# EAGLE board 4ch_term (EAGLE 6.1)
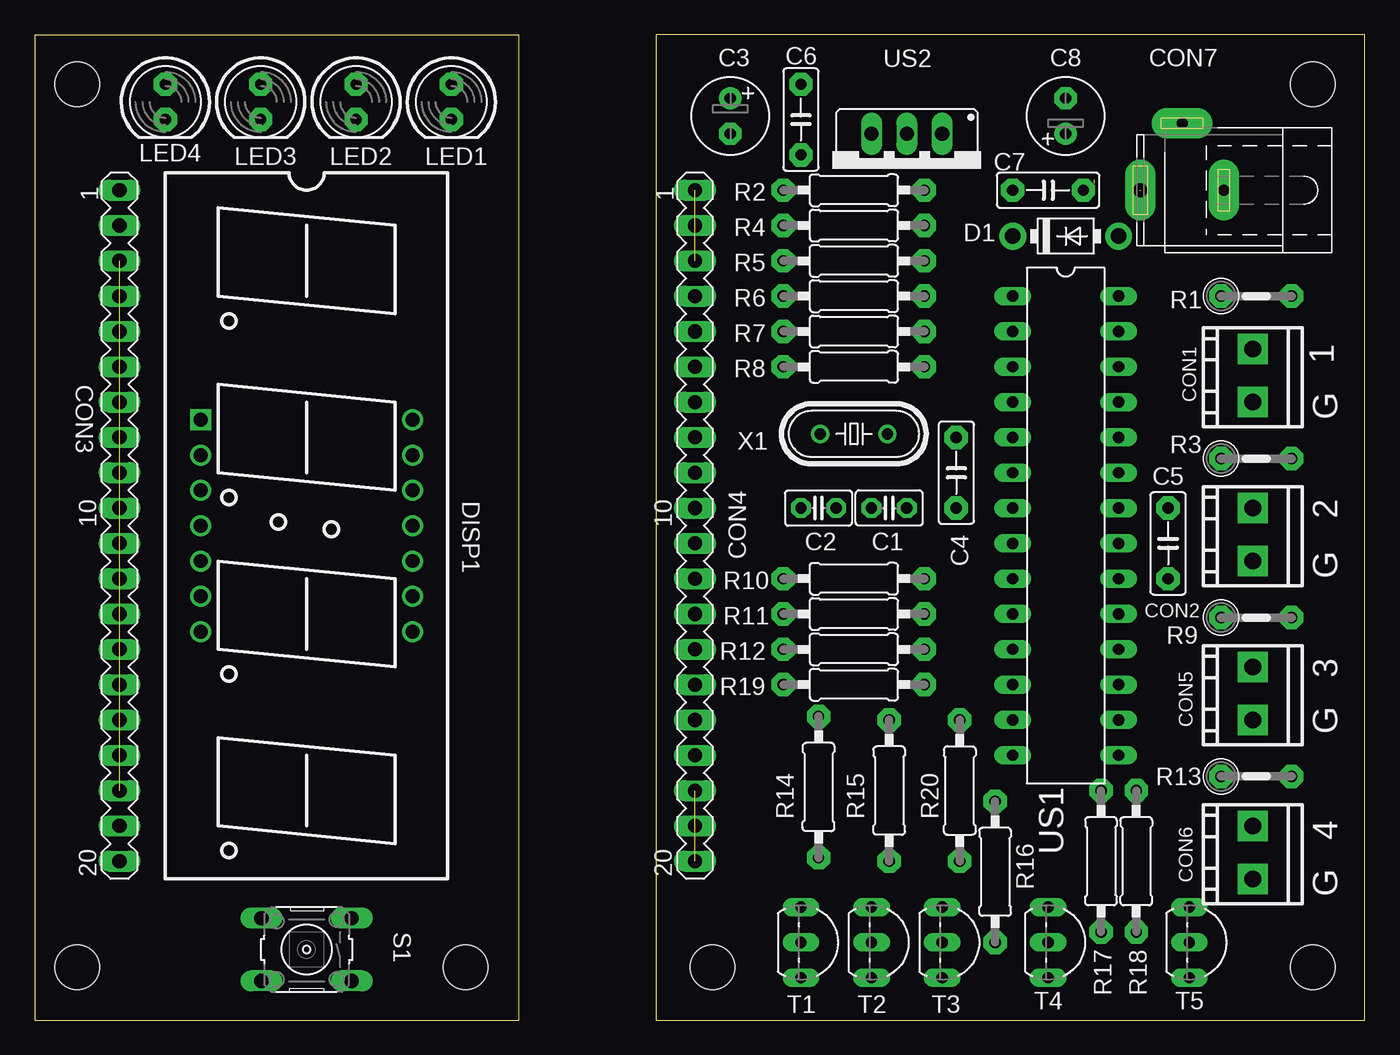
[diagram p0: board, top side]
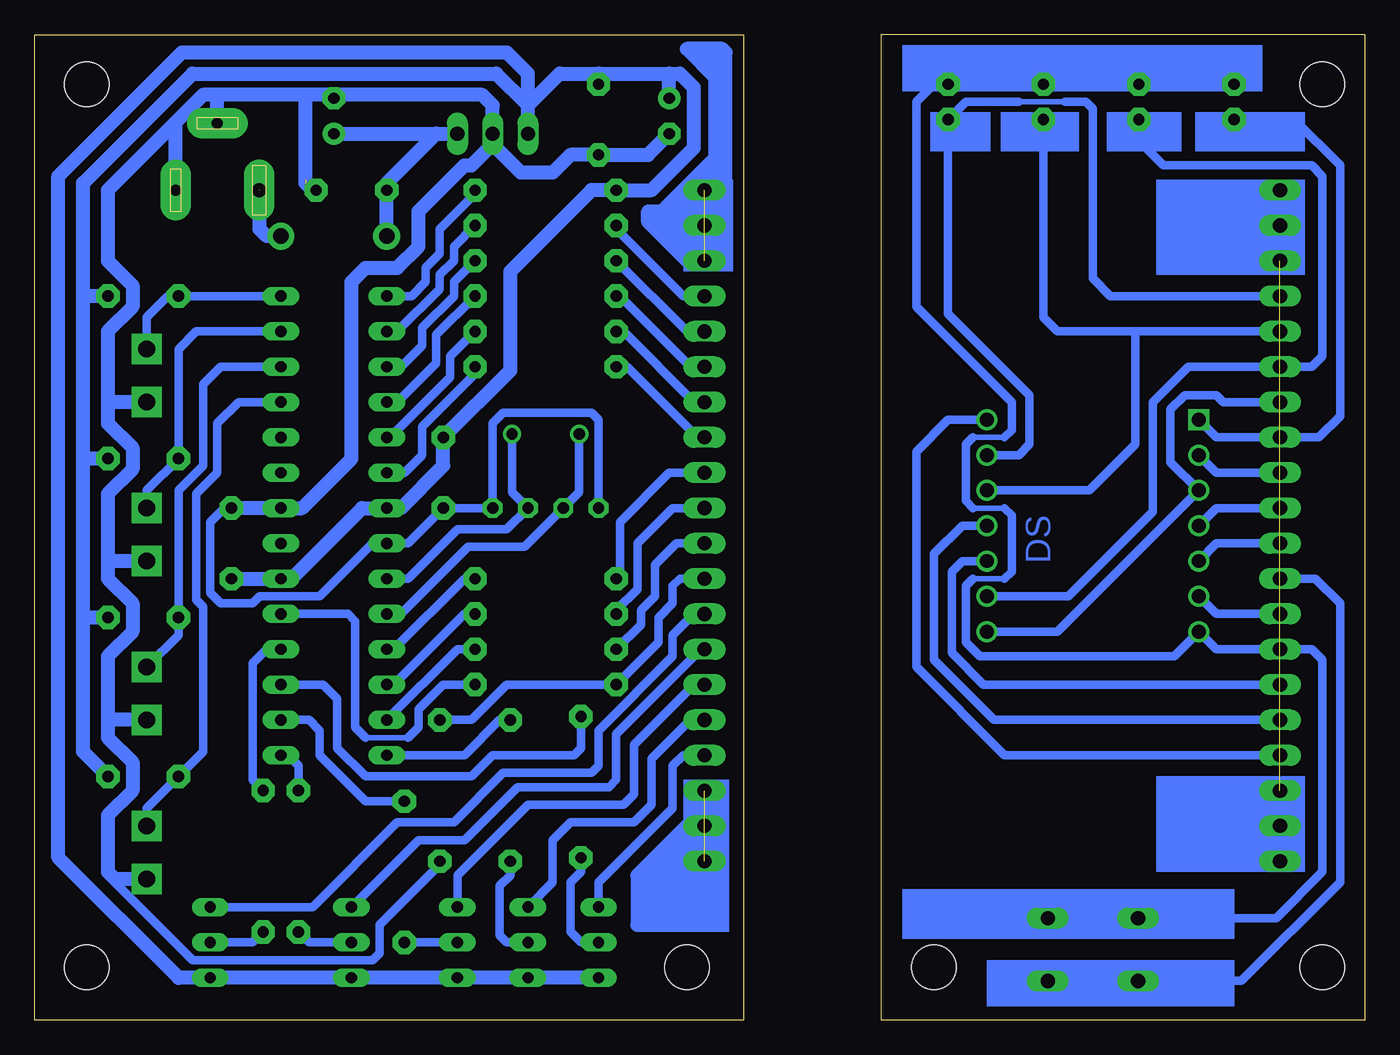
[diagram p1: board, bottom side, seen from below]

Size 95.68 x 70.87 mm. Coordinates in mm from the lower left corner, seen from the top.
Outline: 0,70.86 0,0 34.8,0 34.8,70.86
Outline: 0.01,70.87 34.8,70.87
Outline: 44.7,0 95.68,0 95.68,70.86 44.7,70.86 44.7,0
Copper layers (1*16): Top 0.035mm / dielectric 1.5mm / Bottom 0.035mm
Design rules: minimum track width 10mil, minimum drill 24mil, track to track 8mil, track to pad 8mil, pad to pad 8mil, via to via 8mil, smd to smd 8mil, copper to edge 40mil, drill to drill 8mil, minimum pad ring 10mil, minimum via ring 8mil, stop-mask expansion 4mil, vias tented up to drill 0mil, thermal gap 10mil
Holes 3.2 mm at 91.95,3.81 91.95,67.31 48.77,3.81 3.05,67.31 3.05,3.81 30.99,3.81

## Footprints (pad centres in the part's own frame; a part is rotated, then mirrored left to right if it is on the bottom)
C025-025X050 = drill 0.813 pad 1.422 octagon: 1 -1.27,0; 2 1.27,0
E2,5-6 = drill 0.813 pad 1.6: + -1.27,0 | drill 0.813 pad 1.6 octagon: - 1.27,0
C050-025X075 = drill 0.813 pad 1.676 octagon: 1 -2.54,0; 2 2.54,0
ARK2/300 = drill 1.2 pad 2.184 square: 1 -2.54,0; 2 1.27,0
MA20-1 = drill 1.016 long: 1 -24.13,0; 2 -21.59,0; 3 -19.05,0; 4 -16.51,0; 5 -13.97,0; 6 -11.43,0; 7 -8.89,0; 8 -6.35,0; 9 -3.81,0; 10 -1.27,0; 11 1.27,0; 12 3.81,0; 13 6.35,0; 14 8.89,0; 15 11.43,0; 16 13.97,0; 17 16.51,0; 18 19.05,0; 19 21.59,0; 20 24.13,0
SPC4077 = drill 0.8 pad 2.184 long: 1 -3,0; 2 0,-4.8 | drill 1 pad 2.184 long: 3 3,0
DO41-10 = drill 1.118 pad 1.93: A 3.81,0; C -3.81,0
DISP7X4 = drill 1 square: 1 -7.62,-7.62 | drill 1: 2 -5.08,-7.62; 3 -2.54,-7.62; 4 0,-7.62; 5 2.54,-7.62; 6 5.08,-7.62; 7 7.62,-7.62; 8 7.62,7.62; 9 5.08,7.62; 10 2.54,7.62; 11 0,7.62; 12 -2.54,7.62; 13 -5.08,7.62; 14 -7.62,7.62
LED5MM = drill 0.813 pad 1.676 octagon: A -1.27,0; K 1.27,0
0207/5V = drill 0.813 pad 1.676 octagon: 1 -2.54,0; 2 2.54,0
0207/10 = drill 0.813 pad 1.676 octagon: 1 -5.08,0; 2 5.08,0
B3F-10XX = drill 1.016 long: 1 -3.251,2.261; 2 3.251,2.261; 3 -3.251,-2.261; 4 3.251,-2.261
TO92-EBC = drill 0.813 long: B 0,-1.27; C -2.54,-1.27; E 2.54,-1.27
DIL28-3 = drill 0.813 long: 1 -16.51,-3.81; 2 -13.97,-3.81; 3 -11.43,-3.81; 4 -8.89,-3.81; 5 -6.35,-3.81; 6 -3.81,-3.81; 7 -1.27,-3.81; 8 1.27,-3.81; 9 3.81,-3.81; 10 6.35,-3.81; 11 8.89,-3.81; 12 11.43,-3.81; 13 13.97,-3.81; 14 16.51,-3.81; 15 16.51,3.81; 16 13.97,3.81; 17 11.43,3.81; 18 8.89,3.81; 19 6.35,3.81; 20 3.81,3.81; 21 1.27,3.81; 22 -1.27,3.81; 23 -3.81,3.81; 24 -6.35,3.81; 25 -8.89,3.81; 26 -11.43,3.81; 27 -13.97,3.81; 28 -16.51,3.81
78XXS = drill 1.016 long: GND 0,-2.54; IN -2.54,-2.54; OUT 2.54,-2.54
HC49/S = drill 0.813: 1 -2.413,0; 2 2.413,0

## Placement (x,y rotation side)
C1  [C025-025X050]  61.47,36.83 180 top
C2  [C025-025X050]  56.39,36.83 0 top
C3  220uF  [E2,5-6]  50.04,65.02 270 top
C4  100n  [C050-025X075]  66.29,39.37 270 top
C5  100n  [C050-025X075]  81.53,34.29 90 top
C6  100n  [C050-025X075]  55.12,64.77 270 top
C7  100n  [C050-025X075]  72.9,59.69 0 top
C8  220uF  [E2,5-6]  74.17,65.02 90 top
CON1  [ARK2/300]  87.63,46.99 90 top
CON2  [ARK2/300]  87.63,35.56 90 top
CON3  [MA20-1]  6.1,35.56 270 top
CON4  [MA20-1]  47.5,35.56 270 top
CON5  [ARK2/300]  87.63,24.13 90 top
CON6  [ARK2/300]  87.63,12.7 90 top
CON7  [SPC4077]  82.55,59.69 180 top
D1  1N4004  [DO41-10]  74.17,56.39 0 top
DISP1  DISP7X4  [DISP7X4]  19.56,35.56 270 top
LED1  [LED5MM]  29.97,66.04 270 top
LED2  [LED5MM]  23.11,66.04 270 top
LED3  [LED5MM]  16.26,66.04 270 top
LED4  [LED5MM]  9.4,66.04 270 top
R1  4.7k  [0207/5V]  87.88,52.07 0 top
R2  [0207/10]  58.93,59.69 0 top
R3  4.7k  [0207/5V]  87.88,40.39 0 top
R4  [0207/10]  58.93,57.15 0 top
R5  [0207/10]  58.93,54.61 0 top
R6  [0207/10]  58.93,52.07 0 top
R7  [0207/10]  58.93,49.53 0 top
R8  [0207/10]  58.93,46.99 0 top
R9  4.7k  [0207/5V]  87.88,28.96 0 top
R10  [0207/10]  58.93,31.75 0 top
R11  [0207/10]  58.93,29.21 0 top
R12  [0207/10]  58.93,26.67 0 top
R13  4.7k  [0207/5V]  87.88,17.53 0 top
R14  [0207/10]  56.39,16.76 90 top
R15  [0207/10]  61.47,16.51 90 top
R16  [0207/10]  69.09,10.67 90 top
R17  [0207/10]  76.71,11.43 90 top
R18  [0207/10]  79.25,11.43 90 top
R19  [0207/10]  58.93,24.13 0 top
R20  [0207/10]  66.55,16.51 270 top
S1  [B3F-10XX]  19.56,5.08 180 top
T1  [TO92-EBC]  56.39,5.59 270 top
T2  [TO92-EBC]  61.47,5.59 270 top
T3  [TO92-EBC]  66.55,5.59 270 top
T4  [TO92-EBC]  74.17,5.59 270 top
T5  [TO92-EBC]  84.33,5.59 270 top
US1  ATMEGA8  [DIL28-3]  74.17,35.56 270 top
US2  7805  [78XXS]  62.74,61.21 180 top
X1  8MHz  [HC49/S]  58.93,42.16 0 top

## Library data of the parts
C1-C8 R1-R20 = rcl
CON1 CON2 CON5 CON6 DISP1 = ds_lib_eagle
CON3 CON4 = con-lstb; OC_FARNELL: unknown; OC_NEWARK: unknown
CON7 = con-jack; OC_FARNELL: unknown; OC_NEWARK: unknown
D1 = diode
LED1-LED4 = led
S1 = switch-omron; MPN: B3F-1000; OC_FARNELL: 176432; OC_NEWARK: 36M3542
T1-T5 = transistor-pnp
US1 = avr-4
US2 = v-reg
X1 = crystal; OC_FARNELL: 1667008; OC_NEWARK: unknown

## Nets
+5V: C3.+ C4.1 C5.1 C6.1 R1.2 R2.1 R3.2 R9.2 R13.2 T1.E T2.E T3.E T4.E T5.E US1.7 US1.20 US2.OUT
A: CON3.4 DISP1.13 LED1.K
A1: CON3.17 DISP1.14
A2: CON3.16 DISP1.11
A3: CON3.15 DISP1.10
A4: CON3.13 DISP1.6
A5: CON3.14 DISP1.7 LED1.A LED2.A LED3.A LED4.A S1.4
B: CON3.6 DISP1.9 LED3.K
C: CON3.10 DISP1.4
D: CON3.9 DISP1.2
DP: CON3.7 DISP1.3 DISP1.8
E: CON3.8 DISP1.1 LED4.K
F: CON3.5 DISP1.12 LED2.K
G: CON3.11 DISP1.5
GND: C1.1 C2.1 C3.- C4.2 C5.2 C6.2 C7.2 C8.- CON1.1 CON2.1 CON5.1 CON6.1 CON7.1 CON7.2 R20.2 US1.8 US1.22 US2.GND
N$1: CON4.4 R4.1
N$2: CON4.5 R5.1
N$3: CON4.6 R6.1
N$4: CON4.7 R7.1
N$5: CON4.8 R8.1
N$6: CON4.9 R10.1
N$7: CON4.10 R11.1
N$8: CON4.11 R12.1
N$9: CON4.13 T5.C
N$10: CON4.14 T4.C
N$11: CON4.15 T3.C
N$12: CON4.16 T2.C
N$13: CON4.17 T1.C
N$14: R14.1 T1.B
N$15: R15.1 T2.B
N$16: R16.1 T3.B
N$17: R18.1 T5.B
N$18: R17.1 T4.B
N$19: CON4.12 R19.1 R20.1
N$20: C7.1 C8.+ D1.C US2.IN
N$21: C1.2 US1.9 X1.2
N$22: C2.2 US1.10 X1.1
N$23: R2.2 US1.1
N$24: CON7.3 D1.A
N$33: US1.23
N$34: CON4.18 CON4.19 CON4.20
N$35: CON4.1 CON4.2 CON4.3
N$36: US1.24
NC: CON3.1 CON3.2 CON3.3 CON3.18 CON3.19 CON3.20
SA: R4.2 US1.2
SB: R5.2 US1.3
SC: R6.2 US1.4
SD: R7.2 US1.5
SDP: R12.2 US1.13
SE: R8.2 US1.6
SF: R10.2 US1.11
SG: R11.2 US1.12
SSW: R19.2 US1.19
SW: CON3.12 S1.2
TA1: R15.2 US1.14
TA2: R17.2 US1.15
TA3: R16.2 US1.16
TA4: R14.2 US1.17
TA5: R18.2 US1.18
TR1: CON1.2 R1.1 US1.28
TR2: CON2.2 R3.1 US1.27
TR3: CON5.2 R9.1 US1.26
TR4: CON6.2 R13.1 US1.25

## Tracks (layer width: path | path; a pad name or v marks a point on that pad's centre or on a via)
+5V
  Bottom 1.016: T1.E T2.E | T2.E 60.45,3.05 | T2.E T3.E T4.E T5.E 85.34,3.05 93.98,11.68 93.98,60.71 85.09,69.6 61.72,69.6 60.2,68.07 US2.OUT 60.2,65.79 | 60.2,65.79 62.48,68.07 84.33,68.07 92.2,60.2 92.2,52.07 | 60.2,65.79 57.91,68.07 55.12,68.07 | 55.12,68.07 50.04,68.07 | 50.04,68.07 49.28,68.07 48.26,67.06 48.26,62.74 51.31,59.69 R2.1 55.63,59.69 61.47,53.85 61.47,46.74 C4.1 66.29,39.88 69.34,36.83 US1.7 72.14,36.83 77.22,31.75 US1.20 C5.1 | C3.+ 50.04,68.07 | C6.1 55.12,68.07 | R1.2 92.2,52.07 | R13.2 92.2,19.3 92.2,28.7 | 92.2,28.7 92.2,40.39 | 92.2,40.39 92.2,52.07 | R3.2 92.2,40.39 | R9.2 91.95,28.96 92.2,28.7
A
  Bottom 0.406: 21.59,66.04 24.89,66.04
  Bottom 0.61: DISP1.13 24.89,40.64 24.13,41.4 24.13,44.96 29.97,50.8 LED1.K 28.7,66.04 24.89,66.04 | CON3.4 18.29,52.07 19.56,53.34 19.56,65.53 20.07,66.04 21.59,66.04
A1
  Bottom 0.61: DISP1.14 29.97,43.18 32.26,40.89 32.26,25.4 25.91,19.05 CON3.17
A2
  Bottom 0.61: DISP1.11 28.96,35.56 30.99,33.53 30.99,25.91 26.67,21.59 CON3.16
A3
  Bottom 0.61: DISP1.10 28.96,33.02 29.72,32.26 29.72,26.42 27.43,24.13 CON3.15
A4
  Bottom 0.61: CON3.13 10.67,29.21 DISP1.6
A5
  Bottom 0.406: 28.19,31.75 25.91,31.75 | 25.91,36.83 28.19,36.83 | 28.19,41.91 25.91,41.91
  Bottom 0.61: 28.19,31.75 28.7,31.24 28.7,27.18 27.69,26.16 13.72,26.16 DISP1.7 10.67,26.67 CON3.14 3.81,26.67 3.05,25.91 3.05,10.67 6.38,7.34 S1.4 | 25.91,31.75 25.4,32.26 25.4,36.32 25.91,36.83 | 28.19,36.83 28.7,37.34 28.7,41.4 28.19,41.91 | 25.91,41.91 25.4,42.42 25.4,44.45 32.26,51.31 32.26,66.04 30.99,67.31 LED1.A LED2.A LED3.A LED4.A
B
  Bottom 0.61: DISP1.9 21.34,30.48 15.24,36.58 15.24,44.45 12.7,46.99 CON3.6 3.81,46.99 3.05,47.75 3.05,60.71 3.81,61.47 14.48,61.47 16.26,63.25 LED3.K
C
  Bottom 0.61: CON3.10 10.67,36.83 DISP1.4
D
  Bottom 0.61: CON3.9 10.67,39.37 DISP1.2
DP
  Bottom 0.61: DISP1.8 22.1,27.94 DISP1.3 13.97,40.13 13.97,43.94 12.95,44.96 10.67,44.96 10.16,44.45 CON3.7
E
  Bottom 0.61: DISP1.1 10.67,41.91 CON3.8 3.3,41.91 1.78,43.43 1.78,61.47 5.08,64.77 LED4.K
F
  Bottom 0.61: DISP1.12 19.81,38.1 16.51,41.4 16.51,49.53 | 16.51,49.53 CON3.5 | LED2.K 23.11,50.55 22.1,49.53 16.51,49.53
G
  Bottom 0.61: CON3.11 10.67,34.29 DISP1.5
GND  (1 unrouted)
  Bottom 0.61: C2.1 55.12,43.18 55.63,43.69 61.98,43.69 62.74,42.93 C1.1 C4.2 68.83,34.29 US1.8 71.37,34.29 75.18,30.48 79.5,30.48 80.01,29.97 82.3,29.97 83.06,30.73 83.06,35.81 82.04,36.83 C5.2 | R20.2 66.55,11.18 70.87,6.86 70.87,4.83 71.37,4.32 84.33,4.32 90.42,10.41 90.17,10.41
  Bottom 1.016: 74.17,66.55 63.5,66.55 62.74,65.79 US2.GND 62.74,62.99 | 74.17,66.55 75.95,66.55 | 75.95,66.55 82.55,66.55 | 82.55,66.55 83.57,66.55 85.55,64.56 | 85.55,64.56 90.42,59.69 90.42,54.61 88.65,52.83 88.65,51.31 90.42,49.53 90.42,44.45 | 90.42,44.45 90.42,42.93 88.65,41.15 88.65,39.62 90.42,37.85 90.42,33.02 | 90.42,33.02 90.42,31.75 88.65,29.97 88.65,27.94 90.42,26.16 90.42,21.59 | 90.42,21.59 90.42,20.32 88.65,18.54 88.65,16.51 90.42,14.73 90.42,10.67 90.17,10.41 89.92,10.16 CON6.1 | CON5.1 90.42,21.59 | CON2.1 90.42,33.02 | CON1.1 90.42,44.45 | C8.- 74.17,66.55 | CON7.2 82.55,66.55 | CON7.1 85.55,64.56 | 76.2,60.45 76.2,66.29 75.95,66.55 | C3.- 51.56,62.23 C6.2 57.15,62.23 58.42,60.96 60.71,60.96 62.74,62.99 | C5.2 US1.22 76.45,36.83 72.9,40.39 72.9,53.09 71.88,54.1 69.6,54.1 68.07,55.63 68.07,58.17 64.77,61.47 64.26,61.47 62.74,62.99 | C7.2 75.69,59.69 76.2,60.2
N$1
  Bottom 0.61: R4.1 53.85,56.9 53.59,56.64 49.02,52.07 CON4.4
N$2
  Bottom 0.61: R5.1 48.77,49.53 CON4.5
N$3
  Bottom 0.61: R6.1 53.59,52.07 48.51,46.99 CON4.6
N$4
  Bottom 0.61: R7.1 53.34,49.53 48.26,44.45 CON4.7
N$5
  Bottom 0.61: R8.1 53.09,46.99 48.01,41.91 CON4.8
N$6
  Bottom 0.61: R10.1 53.59,32 53.59,35.81 50.04,39.37 CON4.9
N$7
  Bottom 0.61: CON4.10 49.78,36.83 52.32,34.29 52.32,30.99 53.85,29.46 R11.1
N$8
  Bottom 0.61: CON4.11 49.53,34.29 51.05,32.77 51.05,30.48 52.07,29.46 52.07,28.45 R12.1
N$9
  Bottom 0.61: CON4.13 48.26,29.21 49.78,27.69 49.78,26.16 55.12,20.83 55.12,18.29 55.63,17.78 61.98,17.78 65.53,14.22 69.6,14.22 75.69,8.13 T5.C
N$10
  Bottom 0.61: CON4.14 47.75,26.67 53.85,20.57 53.85,17.27 54.36,16.76 60.96,16.76 64.77,12.95 68.07,12.95 T4.C
N$11
  Bottom 0.61: CON4.15 48.26,24.13 52.58,19.81 52.58,16.26 53.34,15.49 60.2,15.49 65.28,10.41 T3.C
N$12
  Bottom 0.61: CON4.16 48.51,21.59 51.31,18.8 51.31,15.49 52.58,14.22 57.15,14.22 58.42,12.95 58.42,9.91 T2.C
N$13
  Bottom 0.61: CON4.17 49.02,19.05 49.78,18.29 49.78,15.24 55.12,9.91 T1.C
N$14
  Bottom 0.61: R14.1 56.39,10.67 57.15,9.91 57.15,6.35 56.39,5.59 T1.B
N$15
  Bottom 0.61: R15.1 61.47,10.41 62.23,9.65 62.23,6.1 61.72,5.59 T2.B
N$16
  Bottom 0.61: T3.B R16.1
N$17
  Bottom 0.61: T5.B 80.01,5.59 R18.1
N$18
  Bottom 0.61: T4.B 75.95,5.59 R17.1
N$19
  Bottom 0.61: CON4.12 49.28,31.75 49.78,31.24 49.78,29.97 50.8,28.96 50.8,27.18 R19.1 61.72,24.13 64.26,21.59 R20.1
N$20
  Bottom 1.016: C8.+ 66.8,63.75 | 66.8,63.75 US2.IN | D1.C C7.1 70.36,60.2 66.8,63.75
N$21
  Bottom 0.61: X1.2 61.34,37.97 C1.2 61.72,35.31 65.28,35.31 68.83,31.75 US1.9
N$22
  Bottom 0.61: X1.1 56.52,37.97 C2.2 60.45,34.04 64.52,34.04 69.34,29.21 US1.10
N$23
  Bottom 0.61: R2.2 64.01,59.44 66.55,56.9 66.55,55.12 67.56,54.1 67.56,53.09 68.58,52.07 US1.1 70.61,52.07
N$24  (1 unrouted)
  Bottom 1.016: D1.A 78.99,56.39 79.5,56.9 79.5,59.69
N$25
  Bottom 0.61: 16.26,7.37 22.86,7.37
N$26
  Bottom 0.61: 16.26,2.79 22.86,2.79
N$27
  Bottom 1.016: 48.26,14.48 52.32,10.41 52.32,6.86 48.77,6.86
N$28
  Bottom 1.016: 48.51,54.36 51.56,57.4 51.56,58.17 50.29,58.17 48.77,59.69 48.26,59.69
N$29
  Bottom 1.016: 50.8,57.66 49.02,55.88
N$30
  Bottom 1.016: 50.04,58.17 48.77,56.9
N$31
  Bottom 1.016: 49.02,58.93 49.28,58.67 49.28,57.91
N$32
  Bottom 1.016: 45.97,60.2 45.97,69.6 46.23,69.85 48.77,69.85 46.74,67.82 46.74,61.98 50.55,58.17 50.55,57.91
N$34  (2 unrouted)
N$35  (2 unrouted)
N$37
  Bottom 1.016: 46.48,61.47 47.24,60.71 47.24,60.45 46.48,60.45
N$38
  Bottom 1.016: 46.74,69.34 46.48,69.09 46.48,68.58 47.24,69.34
NC  (1 unrouted)
  Bottom 0.61: CON3.1 CON3.2 CON3.3 | CON3.18 CON3.19 CON3.20
SA
  Bottom 0.61: US1.2 69.6,49.53 66.55,52.58 66.55,53.59 65.53,54.61 65.53,55.63 R4.2
SB
  Bottom 0.61: US1.3 69.34,46.99 67.82,48.51 67.82,49.78 65.53,52.07 65.53,53.09 R5.2
SC
  Bottom 0.61: US1.4 69.6,44.45 66.8,47.24 66.8,49.28 R6.2
SD
  Bottom 0.61: US1.5 70.1,41.91 65.79,46.23 65.79,47.75 R7.2
SDP
  Bottom 0.61: US1.13 65.28,26.67 R12.2
SE
  Bottom 0.61: R8.2 64.01,46.48 67.82,42.67 67.82,40.64 69.09,39.37 US1.6 70.61,39.37
SF
  Bottom 0.61: US1.11 69.85,26.67 64.77,31.75 R10.2
SG
  Bottom 0.61: US1.12 69.85,24.13 64.77,29.21 R11.2
SSW
  Bottom 0.406: 68.83,20.32 71.88,20.32
  Bottom 0.61: R19.2 66.29,24.13 68.07,22.35 68.07,21.08 68.83,20.32 | US1.19 73.15,29.21 72.64,28.7 72.64,21.08 71.88,20.32
SW
  Bottom 0.61: S1.2 8.86,2.82 1.78,9.91 1.78,29.97 3.56,31.75 CON3.12
TA1
  Bottom 0.61: R15.2 62.23,21.59 64.77,19.05 US1.14
TA2
  Bottom 0.61: US1.15 77.47,19.05 76.71,18.29 R17.2
TA3
  Bottom 0.61: US1.16 75.95,21.59 75.18,20.83 75.18,19.05 71.88,15.75 R16.2
TA4
  Bottom 0.61: R14.2 56.39,19.56 56.9,19.05 62.74,19.05 64.26,17.53 71.88,17.53 73.91,19.56 73.91,23.11 74.93,24.13 US1.17
TA5
  Bottom 0.61: US1.18 78.99,26.67 80.01,25.65 80.01,17.27 R18.2
TR1
  Bottom 0.61: CON1.2 87.63,50.55 86.11,52.07 R1.1 US1.28
TR2
  Bottom 0.61: US1.27 84.07,49.53 85.34,48.26 R3.1 87.63,38.1 CON2.2
TR3
  Bottom 0.61: US1.26 82.3,46.99 83.57,45.72 83.57,39.88 85.34,38.1 R9.1 85.34,27.69 CON5.2
TR4
  Bottom 0.61: US1.25 81.03,44.45 82.55,42.93 82.55,39.37 84.07,37.85 84.07,30.23 83.57,29.72 83.57,19.3 R13.1 87.63,15.24 CON6.2
(copper drawn outside any net)
  shapes: Bottom area x15

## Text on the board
Bottom: DS
tPlace: 1 | G | 2 | G | 3 | G | 4 | G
